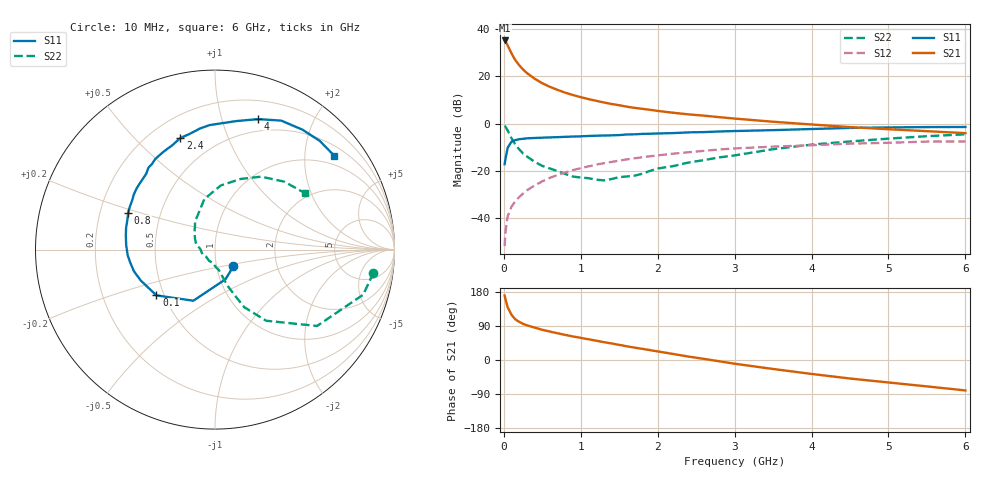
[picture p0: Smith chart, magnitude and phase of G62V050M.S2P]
! SIEMENS Small Signal Semiconductors
! BFG193
! Si NPN RF Bipolar Junction Transistor in SOT223
! VCE = 2 V  IC = 50 mA
! Common Emitter S-Parameters:  August  1996
# GHz  S  MA  R  50
!  f  S11  S21  S12  S22
! GHz  MAG  ANG  MAG  ANG  MAG  ANG  MAG  ANG
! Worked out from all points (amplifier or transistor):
!   36 points, 10 MHz to 6 GHz, reference 50 ohm
!   highest |S21| = 35.0 dB at 10 MHz (marker M1)
!   |S21| within 3 dB of that: start of sweep to 62.99 MHz
!   unconditionally stable (mu >= 1): 368.4 MHz to 2.564 GHz
!   at 250 MHz: K = 0.94, MSG = 26.1 dB, |S12| = -29.5 dB
!   at 1.4 GHz: K = 1.06, MAG = 10.7 dB, |S12| = -16.2 dB
!   at 6 GHz: K = 0.93, MSG = 1.7 dB, |S12| = -7.6 dB
!   S11 on the Smith chart (normalised r, x): 10 MHz: 1.20, -0.23; 100 MHz: 0.45, -0.28; 800 MHz: 0.32, +0.18; 2.4 GHz: 0.32, +0.69; 4 GHz: 0.37, +1.32; 6 GHz: 0.74, +2.72
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0.01  0.1387 -42.7  56.37 170.1  0.0026 83.3  0.8922 -8.3
0.02  0.1753 -70.5  54.05 161.4  0.005 77.5  0.8632 -16.9
0.05  0.3094 -113.0  44.1 139.1  0.0112 68.5  0.7103 -36.8
0.1  0.4143 -142.0  30.01 119.1  0.0177 64.3  0.488 -54.3
0.15  0.4478 -157.3  21.61 107.2  0.023 65.1  0.3596 -63.1
0.2  0.4674 -165.0  16.93 100.6  0.0282 66.7  0.2855 -66.2
0.25  0.4772 -171.0  13.75 95.4  0.0334 66.9  0.2331 -69.4
0.3  0.4874 -176.1  11.6 91.5  0.0391 67.9  0.2021 -71.5
0.4  0.4955 177.1  8.811 85.5  0.0494 68.0  0.156 -74.6
0.5  0.5036 170.6  7.073 79.7  0.0606 67.2  0.128 -77.0
0.6  0.5098 166.3  5.931 75.0  0.0718 66.3  0.1125 -80.6
0.8  0.5253 157.1  4.46 66.2  0.0931 62.8  0.0862 -92.5
1.1  0.547 145.7  3.276 54.7  0.125 57.5  0.0705 -117.5
1.3  0.5582 138.7  2.779 47.1  0.146 53.3  0.0633 -140.4
1.6  0.5883 129.1  2.264 36.1  0.1757 46.2  0.0767 -169.2
2.2  0.6284 112.2  1.687 16.0  0.2314 32.1  0.1266 151.6
2.4  0.6508 107.3  1.561 9.0  0.2481 27.8  0.1505 139.4
3.5  0.7254 80.7  1.091 -23.7  0.3262 0.2  0.2877 101.9
4  0.7664 71.6  0.954 -36.8  0.3482 -9.7  0.3591 84.8
4.5  0.8078 62.8  0.841 -48.9  0.3767 -19.9  0.4189 70.0
5.5  0.8411 46.1  0.69 -69.7  0.4162 -43.1  0.5408 44.4
6  0.8458 38.1  0.627 -80.3  0.4191 -56.2  0.592 32.1
